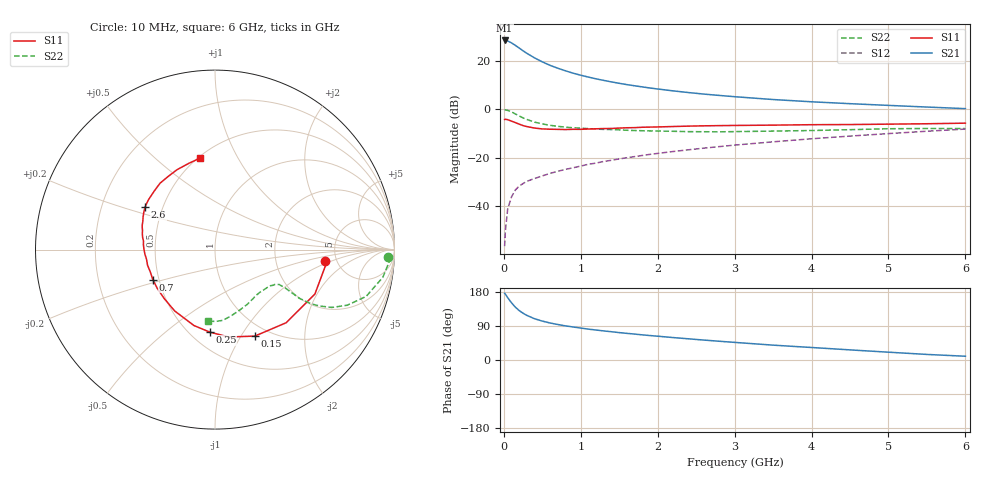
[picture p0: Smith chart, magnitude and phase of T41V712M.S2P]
! Infineon Technologies  Discrete & RF Semiconductors
! BFR182T
! Si NPN RF Bipolar Junction Transistor in SC75
! VCE = 1.75 V  IC = 12 mA
! Common Emitter S-Parameters:  October  1999
# GHz  S  MA  R  50
!  f  S11  S21  S12  S22
! GHz  MAG  ANG  MAG  ANG  MAG  ANG  MAG  ANG
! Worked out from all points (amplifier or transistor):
!   36 points, 10 MHz to 6 GHz, reference 50 ohm
!   highest |S21| = 28.4 dB at 10 MHz (marker M1)
!   |S21| within 3 dB of that: start of sweep to 194 MHz
!   unconditionally stable (mu >= 1): 800.4 MHz to 3.797 GHz
!   at 250 MHz: K = 0.53, MSG = 27.4 dB, |S12| = -30.6 dB
!   at 1.4 GHz: K = 1.11, MAG = 14.1 dB, |S12| = -21.0 dB
!   at 6 GHz: K = 0.85, MSG = 4.2 dB, |S12| = -8.2 dB
!   S11 on the Smith chart (normalised r, x): 10 MHz: 4.02, -0.83; 150 MHz: 0.86, -1.15; 250 MHz: 0.62, -0.72; 700 MHz: 0.46, -0.18; 2.6 GHz: 0.40, +0.24; 6 GHz: 0.51, +0.71
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0.01  0.6154 -6.0  26.23 175.9  0.0015 77.2  0.9647 -2.6
0.02  0.6215 -8.5  26.16 173.9  0.0031 90.7  0.9741 -3.8
0.05  0.6092 -24.0  25.55 164.5  0.0088 82.1  0.9475 -9.4
0.1  0.5685 -45.8  23.36 150.9  0.0156 71.1  0.8818 -17.2
0.15  0.5305 -65.3  20.76 139.3  0.0217 65.0  0.7994 -22.8
0.2  0.4928 -81.1  18.29 130.4  0.026 63.0  0.7273 -26.3
0.25  0.4603 -93.7  16.05 123.4  0.0294 59.0  0.6635 -28.3
0.3  0.4391 -105.5  14.21 117.6  0.0327 58.5  0.6153 -29.4
0.4  0.4089 -123.4  11.44 108.8  0.0373 58.1  0.5418 -30.0
0.5  0.3931 -135.9  9.493 102.7  0.0422 59.2  0.4983 -29.4
0.6  0.3874 -146.2  8.055 97.7  0.0475 60.2  0.4669 -29.0
0.7  0.3846 -154.3  7.024 93.7  0.0525 62.2  0.444 -28.6
0.9  0.3858 -167.0  5.55 87.1  0.062 64.1  0.4146 -28.6
1.1  0.3914 -176.4  4.602 81.4  0.0733 65.6  0.3979 -29.2
1.3  0.3999 176.0  3.932 76.7  0.0839 66.4  0.3841 -30.5
1.6  0.4151 167.3  3.222 70.3  0.1001 67.3  0.3688 -33.0
2.2  0.4403 155.4  2.394 59.2  0.1343 67.6  0.351 -40.4
2.6  0.4552 148.8  2.056 52.6  0.1577 67.0  0.3436 -46.0
3.5  0.4703 135.9  1.586 39.2  0.2128 64.1  0.3543 -59.7
4.5  0.4836 123.0  1.303 26.7  0.2796 59.2  0.379 -75.9
5.5  0.5023 106.9  1.11 14.7  0.3521 53.0  0.4006 -89.7
6  0.5164 99.3  1.03 9.9  0.3901 49.2  0.3993 -95.4
